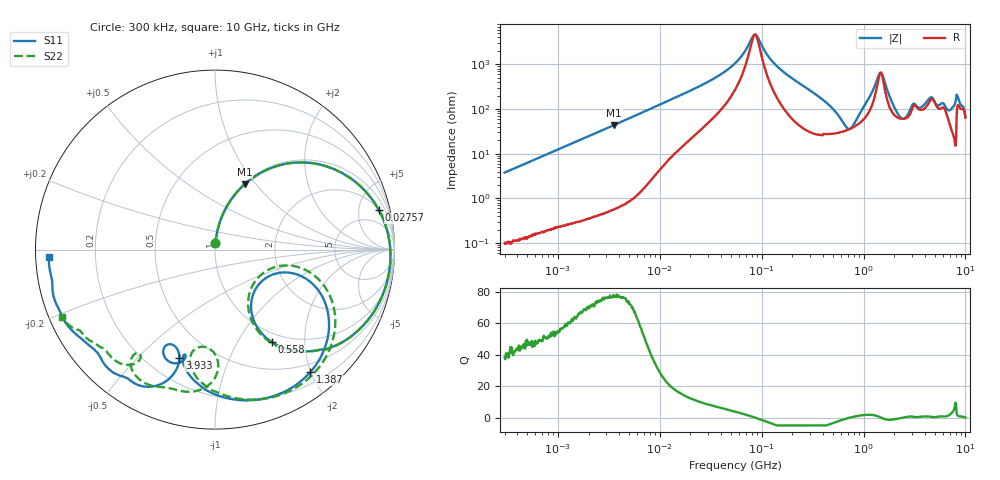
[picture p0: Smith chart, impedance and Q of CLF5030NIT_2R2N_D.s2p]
! S-Parameter Data Generated by TDK Corporation
! Copyright(C) 2019 TDK Corporation.
! All Rights Reserved.
! TDK P/N: CLF5030NIT-2R2N-D (Inductor)
! Property: L=2.2uH at 100kHz
! Size(LxWxT): 5.3x5x2.7mm
! Model Type: s2p (Touchstone File Format Version 1.0)
! Frequency: DC=Yes Start=0.3MHz Stop=10000MHz 802points Log-sweep
! Model Generated on May 10, 2019
! Port Assignments:
!  1 ---@@@--- 2
! Applicable Conditions:
!  Temperature = 25 degC
!  DC Bias Current = 0 A
!  Small Signal Operation
! Terms and conditions regarding TDK Simulation Models
! (1)This simulation model is being provided solely for informational purposes. Please refer to the specifications of the products in terms of detailed characteristics of such products.
! (2)In no event shall TDK Corporation of any of its subsidiaries be liable for any loss or damage arising, directly or indirectly,
!  From any information contained in this simulation model, including, but not limited to loss or damages arising from any inaccuracies, omissions or errors in connection with such information.
! (3)Any and all copyrights on this simulation model are owned by TDK Corporation.
!  Duplication or redistribution of this simulation model without prior written permission from TDK Corporation is prohibited.
! (4)This simulation model is subject to any modification or change without any prior notice.
! (5)Neither TDK Corporation nor any of its subsidiaries shall make any warranty, express or implied,
!  Including but not limited to the correctness, implied warranties of merchantability and fitness for a particular purpose with respect to this simulation models.
! (6)The use of this simulation model shall be deemed to have consented to the terms and conditions hereof.
# Hz S MA R 50
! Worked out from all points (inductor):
!   801 points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, 300 kHz to 10 GHz, reference 50 ohm
!   read as one part in series: L = 2 uH near 318.3 kHz
!   highest Q = 77.3 at 3.554 MHz (marker M1), where L = 1.96 uH
!   self-resonance near 86.06 MHz
!   S11 on the Smith chart (normalised r, x): 300 kHz: 1.00, +0.08; 27.57 MHz: 2.12, +7.90; 558 MHz: 0.87, -1.41; 1.387 GHz: 0.37, -1.99; 3.933 GHz: 0.33, -0.67; 10 GHz: 0.04, -0.02
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300000  0.03792 86.4  0.9983 -2.2  0.9981 -2.1  0.03817 86.7
1713600  0.206 77.2  0.9754 -11.9  0.9755 -11.9  0.2061 77.2
3553821  0.3987 65.6  0.9118 -23.6  0.912 -23.6  0.3988 65.6
9671944  0.7594 38.4  0.626 -49.8  0.6262 -49.8  0.7593 38.4
2.756802e7  0.9395 13.5  0.2536 -70.1  0.2536 -70.1  0.9395 13.5
5.477226e7  0.9723 2.9  0.09243 -72.3  0.09247 -72.3  0.9724 2.9
8.740098e7  0.9791 -3.7  0.02109 4.6  0.02109 4.6  0.9792 -3.7
1.454054e8  0.9729 -12.2  0.1125 67.2  0.1126 67.2  0.973 -12.2
3.126428e8  0.8975 -32.8  0.3499 50.6  0.3499 50.5  0.8976 -32.9
5.580434e8  0.6052 -58.4  0.6262 13.1  0.6263 13.1  0.6015 -59.1
7.84152e8  0.3123 -41.2  0.7013 -26.6  0.7015 -26.6  0.2863 -41.0
9.445544e8  0.4568 -16.9  0.6059 -53.5  0.606 -53.5  0.4349 -11.9
1.387199e9  0.8651 -52.2  0.1404 -82.2  0.1404 -82.2  0.869 -46.4
1.525386e9  0.8812 -64.5  0.1095 -36.4  0.1096 -36.4  0.8911 -58.5
1.767019e9  0.8433 -82.3  0.2308 -17.7  0.231 -17.8  0.8612 -76.2
2.507534e9  0.6242 -106.7  0.4104 -67.8  0.4106 -67.9  0.5972 -102.9
3.008786e9  0.6737 -109.9  0.2591 -103.9  0.2589 -104.2  0.6858 -89.0
3.932853e9  0.6363 -108.2  0.216 -119.6  0.2153 -119.4  0.8233 -111.8
4.865898e9  0.8581 -117.2  0.1235 -115.4  0.1244 -115.3  0.7785 -127.0
6.899057e9  0.8753 -141.2  0.1107 -174.1  0.111 -174.1  0.8416 -140.4
8.546531e9  0.9364 -163.8  0.01989 -177.4  0.02001 -177.4  0.9098 -151.9
1e10  0.9258 -177.4  0.01328 -106.5  0.01305 -106.7  0.9286 -156.2
